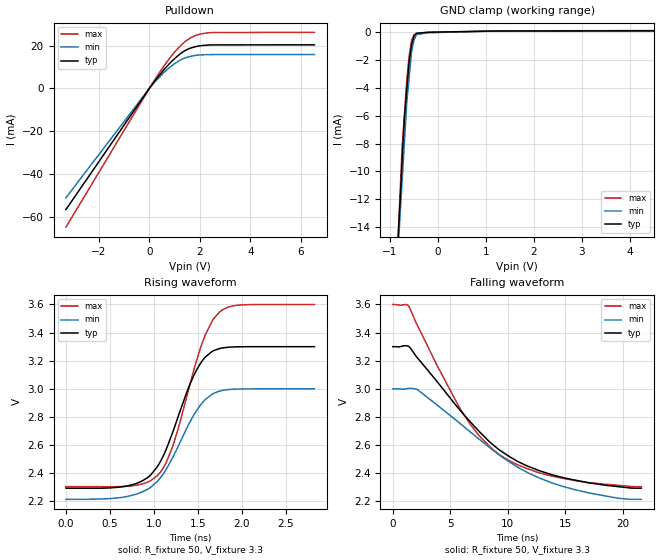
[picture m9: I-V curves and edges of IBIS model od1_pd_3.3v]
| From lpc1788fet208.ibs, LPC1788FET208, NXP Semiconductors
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[Model]   od1_pd_3.3v
Model_type I/O_open_drain
Vinl=8.000E-01
Vinh=2.000E+00
Vref=3.300E+00
Rref=2.000E+03
Cref=0.000E+00
Vmeas=1.650E+00
C_comp   1.240E-12   1.180E-12   1.300E-12
[Voltage Range]   3.300E+00   3.000E+00   3.600E+00
[POWER Clamp Reference]   3.300E+00   3.000E+00   3.600E+00
[GND Clamp Reference]   0.000E+00   0.000E+00   0.000E+00
[Pullup Reference]   3.300E+00   3.000E+00   3.600E+00
[Pulldown Reference]   0.000E+00   0.000E+00   0.000E+00
[Temperature Range]   25   85   -40
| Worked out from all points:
|   slope of the pulldown table from 0 to 0.495 V, typ, clamps not added: 65.7 ohm
|   GND clamp passes 1 mA (typ) near -0.55 V on its own axis
|   rising waveform, R_fixture 50, V_fixture 3.3: 20-80 % time 373ps typ, 403ps min, 362ps max; typ from 2.29 V to 3.3 V
|   falling waveform, R_fixture 50, V_fixture 3.3: 20-80 % time 7.24ns typ, 8.09ns min, 5.99ns max; typ from 3.3 V to 2.29 V
[GND Clamp]
-3.3V     -177.3mA   -158.8mA   -207.6mA
-750mV    -9.48mA    -10.87mA   -8.485mA
-700mV    -6.189mA   -7.965mA   -5.957mA
-650mV    -4.159mA   -5.063mA   -3.43mA
-600mV    -2.128mA   -3.252mA   -1.687mA
-550mV    -914.7uA   -1.441mA   -630.3uA
-500mV    -306.1uA   -590.9uA   -184.3uA
-450mV    -93.32uA   -195.9uA   -156.7uA
-225mV    -19.98uA   -51.54uA   -44.27uA
1.05V     62.05uA    54.96uA    59.19uA
6.6V      98.62uA    85.9uA     109.4uA
[Pulldown]
-3.3V     -56.5mA    -51.02mA   -64.74mA
133mV     2.157mA    1.865mA    2.546mA
552.2mV   8.383mA    7.138mA    10.03mA
791.7mV   11.49mA    9.679mA    13.86mA
1.011V    14.03mA    11.69mA    17.12mA
1.41V     17.6mA     14.25mA    21.79mA
1.65V     18.89mA    15.04mA    23.71mA
1.869V    19.61mA    15.52mA    24.88mA
2.389V    20.29mA    15.78mA    26.03mA
6.54V     20.37mA    15.82mA    26.19mA
[Rising Waveform]
R_fixture = 50
V_fixture = 3.3
V_fixture_min = 3
V_fixture_max = 3.6
0s        2.293V     2.214V     2.304V
725ps     2.314V     2.239V     2.308V
925ps     2.368V     2.285V     2.336V
1.041ns   2.448V     2.343V     2.384V
1.214ns   2.692V     2.512V     2.592V
1.487ns   3.136V     2.848V     3.206V
1.586ns   3.227V     2.925V     3.386V
1.76ns    3.289V     2.986V     3.553V
1.983ns   3.299V     2.999V     3.596V
2.825ns   3.3V       3V         3.6V
[Falling Waveform]
R_fixture = 50
V_fixture = 3.3
V_fixture_min = 3
V_fixture_max = 3.6
0s        3.3V       3V         3.6V
1.373ns   3.302V     3.003V     3.588V
2.147ns   3.219V     2.994V     3.449V
5.968ns   2.836V     2.745V     2.843V
7.541ns   2.694V     2.639V     2.663V
9.139ns   2.573V     2.536V     2.54V
11.5ns    2.458V     2.413V     2.438V
14.66ns   2.371V     2.309V     2.366V
19.05ns   2.309V     2.229V     2.317V
21.6ns    2.293V     2.214V     2.304V
[Ramp]
dV/dt_r   6.0392E-01/3.7240E-10   4.7144E-01/4.0290E-10   7.7735E-01/3.5950E-10
dV/dt_f   6.0392E-01/7.2206E-09   4.7144E-01/8.0847E-09   7.7735E-01/5.9653E-09
R_load = 50
